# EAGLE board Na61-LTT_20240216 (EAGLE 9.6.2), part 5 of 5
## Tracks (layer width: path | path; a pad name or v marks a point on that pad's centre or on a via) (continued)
S$4670 (continued)
  Bottom 0.152: -7.4,145 -7.6,144.8
S$4671
  Bottom 0.152: -7.6,144.8 -7.6,144
S$4672
  Bottom 0.152: -9.4,145 -9.2,144.8
S$4673
  Bottom 0.152: -9.2,144.8 -9.2,144
S$4674
  Bottom 0.152: -11.4,145 -10.8,144.4
S$4675
  Bottom 0.152: -10.8,144.4 -10.8,144
S$4676
  Bottom 0.152: -13.4,145 -12.4,144
S$4677
  Bottom 0.152: -15.4,145 -14.4,144
S$4678
  Bottom 0.152: -14.4,144 -14,144
S$4679
  Bottom 0.152: -17.4,145 -16.4,144
S$4680
  Bottom 0.152: -16.4,144 -15.6,144
S$4681
  Bottom 0.152: -14.6,139 -15.6,140
S$4682
  Bottom 0.152: -15.6,140 -17.2,140
S$4683
  Bottom 0.152: -16.6,139 -17.4,139
S$4684
  Bottom 0.152: -17.4,139 -18.4,140
S$4685
  Bottom 0.152: -18.4,140 -18.8,140
S$4686
  Bottom 0.152: -18.6,139 -19.4,139
S$4687
  Bottom 0.152: -19.4,139 -20.4,140
S$4688
  Bottom 0.152: -20.6,139 -21,139
S$4689
  Bottom 0.152: -21,139 -22,140
S$4690
  Bottom 0.152: -22.6,139 -23.6,140
S$4691
  Bottom 0.152: -24.6,139 -25.2,139.6
S$4692
  Bottom 0.152: -25.2,139.6 -25.2,140
S$4693
  Bottom 0.152: -15.6,143 -16.2,143
S$4694
  Bottom 0.152: -16.2,143 -17.2,144
S$4695
  Bottom 0.152: -17.2,144 -18,144
S$4696
  Bottom 0.152: -17.6,143 -18.2,143
S$4697
  Bottom 0.152: -18.2,143 -19.2,144
S$4698
  Bottom 0.152: -19.2,144 -19.6,144
S$4699
  Bottom 0.152: -19.6,143 -20.2,143
S$4700
  Bottom 0.152: -20.2,143 -21.2,144
S$4701
  Bottom 0.152: -21.6,143 -21.8,143
S$4702
  Bottom 0.152: -21.8,143 -22.8,144
S$4703
  Bottom 0.152: -23.6,143 -24.4,143.8
S$4704
  Bottom 0.152: -24.4,143.8 -24.4,144
S$4705
  Bottom 0.152: 0.4,143 1,143
S$4706
  Bottom 0.152: 1,143 2,144
S$4707
  Bottom 0.152: 2.4,143 2.6,143
S$4708
  Bottom 0.152: 2.6,143 3.6,144
S$4709
  Bottom 0.152: 4.4,143 5.2,143.8
S$4710
  Bottom 0.152: 5.2,143.8 5.2,144
S$4711
  Bottom 0.152: 6.4,143 6.8,143.4
S$4712
  Bottom 0.152: 6.8,143.4 6.8,144
S$4713
  Bottom 0.152: 8.4,143 8.4,144
S$4714
  Bottom 0.152: -1.6,143 -0.6,143
S$4715
  Bottom 0.152: -0.6,143 0.4,144
S$4716
  Bottom 0.152: -0.6,139 0.4,140
S$4717
  Bottom 0.152: 0.4,140 1.2,140
S$4718
  Bottom 0.152: 1.4,139 1.8,139
S$4719
  Bottom 0.152: 1.8,139 2.8,140
S$4720
  Bottom 0.152: 3.4,139 4.4,140
S$4721
  Bottom 0.152: 5.4,139 6,139.6
S$4722
  Bottom 0.152: 6,139.6 6,140
S$4723
  Bottom 0.152: 7.4,139 7.6,139.2
S$4724
  Bottom 0.152: 7.6,139.2 7.6,140
S$4725
  Bottom 0.152: 9.4,139 9.2,139.2
S$4726
  Bottom 0.152: 9.2,139.2 9.2,140
S$4727
  Bottom 0.152: 11.4,139 10.8,139.6
S$4728
  Bottom 0.152: 10.8,139.6 10.8,140
S$4729
  Bottom 0.152: 13.4,139 12.4,140
S$4730
  Bottom 0.152: 15.4,139 15,139
S$4731
  Bottom 0.152: 15,139 14,140
S$4732
  Bottom 0.152: 17.4,139 16.6,139
S$4733
  Bottom 0.152: 16.6,139 15.6,140
S$4734
  Bottom 0.152: 10.4,143 10,143.4
S$4735
  Bottom 0.152: 10,143.4 10,144
S$4736
  Bottom 0.152: 12.4,143 11.6,143.8
S$4737
  Bottom 0.152: 11.6,143.8 11.6,144
S$4738
  Bottom 0.152: 14.4,143 14.2,143
S$4739
  Bottom 0.152: 14.2,143 13.2,144
S$4740
  Bottom 0.152: 16.4,143 15.8,143
S$4741
  Bottom 0.152: 15.8,143 14.8,144
S$4742
  Bottom 0.152: 18.4,141 17.4,140
S$4743
  Bottom 0.152: 17.4,140 16.4,140
S$4744
  Bottom 0.152: 16.6,145 17.2,145
S$4745
  Bottom 0.152: 17.2,145 18.2,144
S$4746
  Bottom 0.152: 18.2,144 18.8,144
S$4747
  Bottom 0.152: 18.6,145 19.6,144
S$4748
  Bottom 0.152: 19.6,144 20.4,144
S$4749
  Bottom 0.152: 20.6,145 21.6,144
S$4750
  Bottom 0.152: 21.6,144 22,144
S$4751
  Bottom 0.152: 22.6,145 23.6,144
S$4752
  Bottom 0.152: 24.6,145 25.2,144.4
S$4753
  Bottom 0.152: 25.2,144.4 25.2,144
S$4754
  Bottom 0.152: 15.6,149 16.6,148
S$4755
  Bottom 0.152: 16.6,148 18,148
S$4756
  Bottom 0.152: 17.6,149 18,149
S$4757
  Bottom 0.152: 18,149 19,148
S$4758
  Bottom 0.152: 19,148 19.6,148
S$4759
  Bottom 0.152: 19.6,149 20.2,149
S$4760
  Bottom 0.152: 20.2,149 21.2,148
S$4761
  Bottom 0.152: 21.6,149 21.8,149
S$4762
  Bottom 0.152: 21.8,149 22.8,148
S$4763
  Bottom 0.152: 23.6,149 24.4,148.2
S$4764
  Bottom 0.152: 24.4,148.2 24.4,148
S$4765
  Bottom 0.152: 17.2,144 16,144
S$4766
  Bottom 0.152: 16,144 15,145
S$4767
  Bottom 0.152: 15,145 14.6,145
S$4768
  Bottom 0.152: 50.8,143 50.2,143
S$4769
  Bottom 0.152: 50.2,143 49.2,144
S$4770
  Bottom 0.152: 48.8,143 48.6,143
S$4771
  Bottom 0.152: 48.6,143 47.6,144
S$4772
  Bottom 0.152: 46.8,143 46,143.8
S$4773
  Bottom 0.152: 46,143.8 46,144
S$4774
  Bottom 0.152: 44.8,143 44.4,143.4
S$4775
  Bottom 0.152: 44.4,143.4 44.4,144
S$4776
  Bottom 0.152: 42.8,143 42.8,144
S$4777
  Bottom 0.152: 52.8,143 51.8,143
S$4778
  Bottom 0.152: 51.8,143 50.8,144
S$4779
  Bottom 0.152: 51.8,139 50.8,140
S$4780
  Bottom 0.152: 50.8,140 50,140
S$4781
  Bottom 0.152: 49.8,139 49.4,139
S$4782
  Bottom 0.152: 49.4,139 48.4,140
S$4783
  Bottom 0.152: 47.8,139 46.8,140
S$4784
  Bottom 0.152: 45.8,139 45.2,139.6
S$4785
  Bottom 0.152: 45.2,139.6 45.2,140
S$4786
  Bottom 0.152: 43.8,139 43.6,139.2
S$4787
  Bottom 0.152: 43.6,139.2 43.6,140
S$4788
  Bottom 0.152: 41.8,139 42,139.2
S$4789
  Bottom 0.152: 42,139.2 42,140
S$4790
  Bottom 0.152: 39.8,139 40.4,139.6
S$4791
  Bottom 0.152: 40.4,139.6 40.4,140
S$4792
  Bottom 0.152: 37.8,139 38.8,140
S$4793
  Bottom 0.152: 35.8,139 36.2,139
S$4794
  Bottom 0.152: 36.2,139 37.2,140
S$4795
  Bottom 0.152: 33.8,139 34.6,139
S$4796
  Bottom 0.152: 34.6,139 35.6,140
S$4797
  Bottom 0.152: 40.8,143 41.2,143.4
S$4798
  Bottom 0.152: 41.2,143.4 41.2,144
S$4799
  Bottom 0.152: 38.8,143 39.6,143.8
S$4800
  Bottom 0.152: 39.6,143.8 39.6,144
S$4801
  Bottom 0.152: 36.8,143 37,143
S$4802
  Bottom 0.152: 37,143 38,144
S$4803
  Bottom 0.152: 34.8,143 35.4,143
S$4804
  Bottom 0.152: 35.4,143 36.4,144
S$4805
  Bottom 0.152: 32.8,141 33.8,140
S$4806
  Bottom 0.152: 33.8,140 34.8,140
S$4807
  Bottom 0.152: 34.6,145 34,145
S$4808
  Bottom 0.152: 34,145 33,144
S$4809
  Bottom 0.152: 33,144 32.4,144
S$4810
  Bottom 0.152: 32.6,145 31.6,144
S$4811
  Bottom 0.152: 31.6,144 30.8,144
S$4812
  Bottom 0.152: 30.6,145 29.6,144
S$4813
  Bottom 0.152: 29.6,144 29.2,144
S$4814
  Bottom 0.152: 28.6,145 27.6,144
S$4815
  Bottom 0.152: 26.6,145 26,144.4
S$4816
  Bottom 0.152: 26,144.4 26,144
S$4817
  Bottom 0.152: 35.6,149 34.6,148
S$4818
  Bottom 0.152: 34.6,148 33.2,148
S$4819
  Bottom 0.152: 33.6,149 33.2,149
S$4820
  Bottom 0.152: 33.2,149 32.2,148
S$4821
  Bottom 0.152: 32.2,148 31.6,148
S$4822
  Bottom 0.152: 31.6,149 31,149
S$4823
  Bottom 0.152: 31,149 30,148
S$4824
  Bottom 0.152: 29.6,149 29.4,149
S$4825
  Bottom 0.152: 29.4,149 28.4,148
S$4826
  Bottom 0.152: 27.6,149 26.8,148.2
S$4827
  Bottom 0.152: 26.8,148.2 26.8,148
S$4828
  Bottom 0.152: 34,144 35.2,144
S$4829
  Bottom 0.152: 35.2,144 36.2,145
S$4830
  Bottom 0.152: 36.2,145 36.6,145
S$4831  (2 unrouted)
  Top 0.813: 65,148.5 65,139.5
  Top 1.8: 66,145.5 64,145.5 | 66,148.5 65,148.5 64,148.5 | 66,142.5 64,142.5 | 66,139.5 65,139.5 64,139.5
S$4832
  Top 1.778: -104.08,140.82 -104.08,142.35
S$4833
  Top 1.778: -104.08,145.65 -104.08,147.18
S$4834
  Top 1.778: -99,140.82 -99,142.35
S$4835
  Top 1.778: -99,145.65 -99,147.18
S$4836
  Top 1.778: -93.92,140.82 -93.92,142.35
S$4837
  Top 1.778: -93.92,145.65 -93.92,147.18
S$4838
  Top 1.778: 93.92,140.82 93.92,142.35
S$4839
  Top 1.778: 93.92,145.65 93.92,147.18
S$4840
  Top 1.778: 99,140.82 99,142.35
S$4841
  Top 1.778: 99,145.65 99,147.18
S$4842
  Top 1.778: 104.08,140.82 104.08,142.35
S$4843
  Top 1.778: 104.08,145.65 104.08,147.18
S$4844  (via drill 0.2)
  other vias: -25.6,150.4
S$4845  (via drill 0.2)
  other vias: -8.6,137.6
S$4846  (via drill 0.2)
  other vias: 8.6,150.4
S$4847  (via drill 0.2)
  other vias: 25.6,137.6
S$4848  (via drill 0.2)
  other vias: 41.6,150.4
S$4849  (via drill 0.2)
  other vias: 52.8,150.4
S$4850  (via drill 0.2)
  other vias: -41.6,137.6
S$4851  (via drill 0.2)
  other vias: -52.8,137.6
S$4852
  Bottom 0.8: 9.4,156.9 9.4,155.1
S$4853
  Bottom 0.8: 11.4,156.9 11.4,155.1
S$4854
  Bottom 0.8: 8.4,159.1 8.4,160.9
S$4855
  Bottom 0.8: 10.4,159.1 10.4,160.9
S$4856
  Bottom 0.8: 5.4,156.9 5.4,155.1
S$4857
  Bottom 0.8: 7.4,156.9 7.4,155.1
S$4858
  Bottom 0.8: 6.4,159.1 6.4,160.9
S$4859
  Bottom 0.8: 4.4,159.1 4.4,160.9
S$4860
  Bottom 0.8: 3.4,156.9 3.4,155.1
S$4861
  Bottom 0.8: 1.4,156.9 1.4,155.1
S$4862
  Bottom 0.8: 2.4,159.1 2.4,160.9
S$4863
  Bottom 0.8: 0.4,159.1 0.4,160.9
S$4864
  Bottom 0.8: -0.6,156.9 -0.6,155.1
S$4865
  Bottom 0.8: -2.6,156.9 -2.6,155.1
S$4866
  Bottom 0.8: -1.6,159.1 -1.6,160.9
S$4867
  Bottom 0.8: 17.4,156.9 17.4,155.1
S$4868
  Bottom 0.8: 19.4,156.9 19.4,155.1
S$4869
  Bottom 0.8: 16.4,159.1 16.4,160.9
S$4870
  Bottom 0.8: 18.4,159.1 18.4,160.9
S$4871
  Bottom 0.8: 13.4,156.9 13.4,155.1
S$4872
  Bottom 0.8: 15.4,156.9 15.4,155.1
S$4873
  Bottom 0.8: 12.4,159.1 12.4,160.9
S$4874
  Bottom 0.8: 14.4,159.1 14.4,160.9
S$4875
  Bottom 0.8: -7.4,164.9 -7.4,163.1
S$4876
  Bottom 0.8: -5.4,164.9 -5.4,163.1
S$4877
  Bottom 0.8: -8.4,167.1 -8.4,168.9
S$4878
  Bottom 0.8: -6.4,167.1 -6.4,168.9
S$4879
  Bottom 0.8: -11.4,164.9 -11.4,163.1
S$4880
  Bottom 0.8: -9.4,164.9 -9.4,163.1
S$4881
  Bottom 0.8: -10.4,167.1 -10.4,168.9
S$4882
  Bottom 0.8: -12.4,167.1 -12.4,168.9
S$4883
  Bottom 0.8: -13.4,164.9 -13.4,163.1
S$4884
  Bottom 0.8: -15.4,164.9 -15.4,163.1
S$4885
  Bottom 0.8: -14.4,167.1 -14.4,168.9
S$4886
  Bottom 0.8: -16.4,167.1 -16.4,168.9
S$4887
  Bottom 0.8: -17.4,164.9 -17.4,163.1
S$4888
  Bottom 0.8: -19.4,164.9 -19.4,163.1
S$4889
  Bottom 0.8: -18.4,167.1 -18.4,168.9
S$4890
  Bottom 0.8: 0.6,164.9 0.6,163.1
S$4891
  Bottom 0.8: 2.6,164.9 2.6,163.1
S$4892
  Bottom 0.8: -0.4,167.1 -0.4,168.9
S$4893
  Bottom 0.8: 1.6,167.1 1.6,168.9
S$4894
  Bottom 0.8: -3.4,164.9 -3.4,163.1
S$4895
  Bottom 0.8: -1.4,164.9 -1.4,163.1
S$4896
  Bottom 0.8: -4.4,167.1 -4.4,168.9
S$4897
  Bottom 0.8: -2.4,167.1 -2.4,168.9
S$4898
  Bottom 0.8: -24.6,156.9 -24.6,155.1
S$4899
  Bottom 0.8: -22.6,156.9 -22.6,155.1
S$4900
  Bottom 0.8: -25.6,159.1 -25.6,160.9
S$4901
  Bottom 0.8: -23.6,159.1 -23.6,160.9
S$4902
  Bottom 0.8: -28.6,156.9 -28.6,155.1
S$4903
  Bottom 0.8: -26.6,156.9 -26.6,155.1
S$4904
  Bottom 0.8: -27.6,159.1 -27.6,160.9
S$4905
  Bottom 0.8: -29.6,159.1 -29.6,160.9
S$4906
  Bottom 0.8: -30.6,156.9 -30.6,155.1
S$4907
  Bottom 0.8: -32.6,156.9 -32.6,155.1
S$4908
  Bottom 0.8: -31.6,159.1 -31.6,160.9
S$4909
  Bottom 0.8: -33.6,159.1 -33.6,160.9
S$4910
  Bottom 0.8: -34.6,156.9 -34.6,155.1
S$4911
  Bottom 0.8: -36.6,156.9 -36.6,155.1
S$4912
  Bottom 0.8: -35.6,159.1 -35.6,160.9
S$4913
  Bottom 0.8: -16.6,156.9 -16.6,155.1
S$4914
  Bottom 0.8: -14.6,156.9 -14.6,155.1
S$4915
  Bottom 0.8: -17.6,159.1 -17.6,160.9
S$4916
  Bottom 0.8: -15.6,159.1 -15.6,160.9
S$4917
  Bottom 0.8: -20.6,156.9 -20.6,155.1
S$4918
  Bottom 0.8: -18.6,156.9 -18.6,155.1
S$4919
  Bottom 0.8: -21.6,159.1 -21.6,160.9
S$4920
  Bottom 0.8: -19.6,159.1 -19.6,160.9
S$4921
  Bottom 0.8: 26.6,164.9 26.6,163.1
S$4922
  Bottom 0.8: 28.6,164.9 28.6,163.1
S$4923
  Bottom 0.8: 25.6,167.1 25.6,168.9
S$4924
  Bottom 0.8: 27.6,167.1 27.6,168.9
S$4925
  Bottom 0.8: 22.6,164.9 22.6,163.1
S$4926
  Bottom 0.8: 24.6,164.9 24.6,163.1
S$4927
  Bottom 0.8: 23.6,167.1 23.6,168.9
S$4928
  Bottom 0.8: 21.6,167.1 21.6,168.9
S$4929
  Bottom 0.8: 20.6,164.9 20.6,163.1
S$4930
  Bottom 0.8: 18.6,164.9 18.6,163.1
S$4931
  Bottom 0.8: 19.6,167.1 19.6,168.9
S$4932
  Bottom 0.8: 17.6,167.1 17.6,168.9
S$4933
  Bottom 0.8: 16.6,164.9 16.6,163.1
S$4934
  Bottom 0.8: 14.6,164.9 14.6,163.1
S$4935
  Bottom 0.8: 15.6,167.1 15.6,168.9
S$4936
  Bottom 0.8: 34.6,164.9 34.6,163.1
S$4937
  Bottom 0.8: 36.6,164.9 36.6,163.1
S$4938
  Bottom 0.8: 33.6,167.1 33.6,168.9
S$4939
  Bottom 0.8: 35.6,167.1 35.6,168.9
S$4940
  Bottom 0.8: 30.6,164.9 30.6,163.1
S$4941
  Bottom 0.8: 32.6,164.9 32.6,163.1
S$4942
  Bottom 0.8: 29.6,167.1 29.6,168.9
S$4943
  Bottom 0.8: 31.6,167.1 31.6,168.9
S$4944
  Bottom 0.8: -41.8,164.9 -41.8,163.1
S$4945
  Bottom 0.8: -39.8,164.9 -39.8,163.1
S$4946
  Bottom 0.8: -42.8,167.1 -42.8,168.9
S$4947
  Bottom 0.8: -40.8,167.1 -40.8,168.9
S$4948
  Bottom 0.8: -45.8,164.9 -45.8,163.1
S$4949
  Bottom 0.8: -43.8,164.9 -43.8,163.1
S$4950
  Bottom 0.8: -44.8,167.1 -44.8,168.9
S$4951
  Bottom 0.8: -46.8,167.1 -46.8,168.9
S$4952
  Bottom 0.8: -47.8,164.9 -47.8,163.1
S$4953
  Bottom 0.8: -49.8,164.9 -49.8,163.1
S$4954
  Bottom 0.8: -48.8,167.1 -48.8,168.9
S$4955
  Bottom 0.8: -50.8,167.1 -50.8,168.9
S$4956
  Bottom 0.8: -51.8,164.9 -51.8,163.1
S$4957
  Bottom 0.8: -53.8,164.9 -53.8,163.1
S$4958
  Bottom 0.8: -52.8,167.1 -52.8,168.9
S$4959
  Bottom 0.8: -33.8,164.9 -33.8,163.1
S$4960
  Bottom 0.8: -31.8,164.9 -31.8,163.1
S$4961
  Bottom 0.8: -34.8,167.1 -34.8,168.9
S$4962
  Bottom 0.8: -32.8,167.1 -32.8,168.9
S$4963
  Bottom 0.8: -37.8,164.9 -37.8,163.1
S$4964
  Bottom 0.8: -35.8,164.9 -35.8,163.1
S$4965
  Bottom 0.8: -38.8,167.1 -38.8,168.9
S$4966
  Bottom 0.8: -36.8,167.1 -36.8,168.9
S$4967
  Bottom 0.8: 43.8,156.9 43.8,155.1
S$4968
  Bottom 0.8: 45.8,156.9 45.8,155.1
S$4969
  Bottom 0.8: 42.8,159.1 42.8,160.9
S$4970
  Bottom 0.8: 44.8,159.1 44.8,160.9
S$4971
  Bottom 0.8: 39.8,156.9 39.8,155.1
S$4972
  Bottom 0.8: 41.8,156.9 41.8,155.1
S$4973
  Bottom 0.8: 40.8,159.1 40.8,160.9
S$4974
  Bottom 0.8: 38.8,159.1 38.8,160.9
S$4975
  Bottom 0.8: 37.8,156.9 37.8,155.1
S$4976
  Bottom 0.8: 35.8,156.9 35.8,155.1
S$4977
  Bottom 0.8: 36.8,159.1 36.8,160.9
S$4978
  Bottom 0.8: 34.8,159.1 34.8,160.9
S$4979
  Bottom 0.8: 33.8,156.9 33.8,155.1
S$4980
  Bottom 0.8: 31.8,156.9 31.8,155.1
S$4981
  Bottom 0.8: 32.8,159.1 32.8,160.9
S$4982
  Bottom 0.8: 51.8,156.9 51.8,155.1
S$4983
  Bottom 0.8: 53.8,156.9 53.8,155.1
S$4984
  Bottom 0.8: 50.8,159.1 50.8,160.9
S$4985
  Bottom 0.8: 52.8,159.1 52.8,160.9
S$4986
  Bottom 0.8: 47.8,156.9 47.8,155.1
S$4987
  Bottom 0.8: 49.8,156.9 49.8,155.1
S$4988
  Bottom 0.8: 46.8,159.1 46.8,160.9
S$4989
  Bottom 0.8: 48.8,159.1 48.8,160.9
S$4990  (via drill 0.2)
  other vias: -50.8,166
S$4991  (via drill 0.2)
  other vias: -49.2,166
S$4992  (via drill 0.2)
  other vias: -47.6,166
S$4993  (via drill 0.2)
  other vias: -46,166
S$4994  (via drill 0.2)
  other vias: -44.4,166
S$4995  (via drill 0.2)
  other vias: -42.8,166
S$4996  (via drill 0.2)
  other vias: -41.2,166
S$4997  (via drill 0.2)
  other vias: -39.6,166
S$4998  (via drill 0.2)
  other vias: -38,166
S$4999  (via drill 0.2)
  other vias: -36.4,166
S$5000  (via drill 0.2)
  other vias: -34.8,166
S$5001  (via drill 0.2)
  other vias: -50,162
S$5002  (via drill 0.2)
  other vias: -48.4,162
S$5003  (via drill 0.2)
  other vias: -46.8,162
S$5004  (via drill 0.2)
  other vias: -45.2,162
S$5005  (via drill 0.2)
  other vias: -43.6,162
S$5006  (via drill 0.2)
  other vias: -42,162
S$5007  (via drill 0.2)
  other vias: -40.4,162
S$5008  (via drill 0.2)
  other vias: -38.8,162
S$5009  (via drill 0.2)
  other vias: -37.2,162
S$5010  (via drill 0.2)
  other vias: -35.6,162
S$5011  (via drill 0.2)
  other vias: -34,158
S$5012  (via drill 0.2)
  other vias: -32.4,158
S$5013  (via drill 0.2)
  other vias: -30.8,158
S$5014  (via drill 0.2)
  other vias: -29.2,158
S$5015  (via drill 0.2)
  other vias: -27.6,158
S$5016  (via drill 0.2)
  other vias: -33.2,162
S$5017  (via drill 0.2)
  other vias: -31.6,162
S$5018  (via drill 0.2)
  other vias: -30,162
S$5019  (via drill 0.2)
  other vias: -28.4,162
S$5020  (via drill 0.2)
  other vias: -26.8,162
S$5021  (via drill 0.2)
  other vias: -26,158
S$5022  (via drill 0.2)
  other vias: -0.4,166
S$5023  (via drill 0.2)
  other vias: -2,166
S$5024  (via drill 0.2)
  other vias: -3.6,166
S$5025  (via drill 0.2)
  other vias: -5.2,166
S$5026  (via drill 0.2)
  other vias: -6.8,166
S$5027  (via drill 0.2)
  other vias: -8.4,166
S$5028  (via drill 0.2)
  other vias: -10,166
S$5029  (via drill 0.2)
  other vias: -11.6,166
S$5030  (via drill 0.2)
  other vias: -13.2,166
S$5031  (via drill 0.2)
  other vias: -14.8,166
S$5032  (via drill 0.2)
  other vias: -16.4,166
S$5033  (via drill 0.2)
  other vias: -1.2,162
S$5034  (via drill 0.2)
  other vias: -2.8,162
S$5035  (via drill 0.2)
  other vias: -4.4,162
S$5036  (via drill 0.2)
  other vias: -6,162
S$5037  (via drill 0.2)
  other vias: -7.6,162
S$5038  (via drill 0.2)
  other vias: -9.2,162
S$5039  (via drill 0.2)
  other vias: -10.8,162
S$5040  (via drill 0.2)
  other vias: -12.4,162
S$5041  (via drill 0.2)
  other vias: -14,162
S$5042  (via drill 0.2)
  other vias: -15.6,162
S$5043  (via drill 0.2)
  other vias: -17.2,158
S$5044  (via drill 0.2)
  other vias: -18.8,158
S$5045  (via drill 0.2)
  other vias: -20.4,158
S$5046  (via drill 0.2)
  other vias: -22,158
S$5047  (via drill 0.2)
  other vias: -23.6,158
S$5048  (via drill 0.2)
  other vias: -18,162
S$5049  (via drill 0.2)
  other vias: -19.6,162
S$5050  (via drill 0.2)
  other vias: -21.2,162
S$5051  (via drill 0.2)
  other vias: -22.8,162
S$5052  (via drill 0.2)
  other vias: -24.4,162
S$5053  (via drill 0.2)
  other vias: -25.2,158
S$5054  (via drill 0.2)
  other vias: 0.4,162
S$5055  (via drill 0.2)
  other vias: 2,162
S$5056  (via drill 0.2)
  other vias: 3.6,162
S$5057  (via drill 0.2)
  other vias: 5.2,162
S$5058  (via drill 0.2)
  other vias: 6.8,162
S$5059  (via drill 0.2)
  other vias: 8.4,162
S$5060  (via drill 0.2)
  other vias: 10,162
S$5061  (via drill 0.2)
  other vias: 11.6,162
S$5062  (via drill 0.2)
  other vias: 13.2,162
S$5063  (via drill 0.2)
  other vias: 14.8,162
S$5064  (via drill 0.2)
  other vias: 16.4,158
S$5065  (via drill 0.2)
  other vias: 1.2,158
S$5066  (via drill 0.2)
  other vias: 2.8,158
S$5067  (via drill 0.2)
  other vias: 4.4,158
S$5068  (via drill 0.2)
  other vias: 6,158
S$5069  (via drill 0.2)
  other vias: 7.6,158
S$5070  (via drill 0.2)
  other vias: 9.2,158
S$5071  (via drill 0.2)
  other vias: 10.8,158
S$5072  (via drill 0.2)
  other vias: 12.4,158
S$5073  (via drill 0.2)
  other vias: 14,158
S$5074  (via drill 0.2)
  other vias: 15.6,158
S$5075  (via drill 0.2)
  other vias: 17.2,162
S$5076  (via drill 0.2)
  other vias: 18.8,162
S$5077  (via drill 0.2)
  other vias: 20.4,162
S$5078  (via drill 0.2)
  other vias: 18,166
S$5079  (via drill 0.2)
  other vias: 19.6,166
S$5080  (via drill 0.2)
  other vias: 21.2,166
S$5081  (via drill 0.2)
  other vias: 22,162
S$5082  (via drill 0.2)
  other vias: 22.8,166
S$5083  (via drill 0.2)
  other vias: 23.6,162
S$5084  (via drill 0.2)
  other vias: 24.4,166
S$5085  (via drill 0.2)
  other vias: 25.2,162
S$5086  (via drill 0.2)
  other vias: 50.8,162
S$5087  (via drill 0.2)
  other vias: 49.2,162
S$5088  (via drill 0.2)
  other vias: 47.6,162
S$5089  (via drill 0.2)
  other vias: 46,162
S$5090  (via drill 0.2)
  other vias: 44.4,162
S$5091  (via drill 0.2)
  other vias: 42.8,162
S$5092  (via drill 0.2)
  other vias: 41.2,162
S$5093  (via drill 0.2)
  other vias: 39.6,162
S$5094  (via drill 0.2)
  other vias: 38,162
S$5095  (via drill 0.2)
  other vias: 36.4,162
S$5096  (via drill 0.2)
  other vias: 34.8,158
S$5097  (via drill 0.2)
  other vias: 50,158
S$5098  (via drill 0.2)
  other vias: 48.4,158
S$5099  (via drill 0.2)
  other vias: 46.8,158
S$5100  (via drill 0.2)
  other vias: 45.2,158
S$5101  (via drill 0.2)
  other vias: 43.6,158
S$5102  (via drill 0.2)
  other vias: 42,158
S$5103  (via drill 0.2)
  other vias: 40.4,158
S$5104  (via drill 0.2)
  other vias: 38.8,158
S$5105  (via drill 0.2)
  other vias: 37.2,158
S$5106  (via drill 0.2)
  other vias: 35.6,158
S$5107  (via drill 0.2)
  other vias: 34,162
S$5108  (via drill 0.2)
  other vias: 32.4,162
S$5109  (via drill 0.2)
  other vias: 30.8,162
S$5110  (via drill 0.2)
  other vias: 33.2,166
S$5111  (via drill 0.2)
  other vias: 31.6,166
S$5112  (via drill 0.2)
  other vias: 30,166
S$5113  (via drill 0.2)
  other vias: 29.2,162
S$5114  (via drill 0.2)
  other vias: 28.4,166
S$5115  (via drill 0.2)
  other vias: 27.6,162
S$5116  (via drill 0.2)
  other vias: 26.8,166
S$5117  (via drill 0.2)
  other vias: 26,162
S$5118
  Bottom 0.152: -52.8,167 -51.8,166
S$5119
  Bottom 0.152: -51.8,166 -50.8,166
S$5120
  Bottom 0.152: -50.8,167 -50.2,167
S$5121
  Bottom 0.152: -50.2,167 -49.2,166
S$5122
  Bottom 0.152: -48.8,167 -48.6,167
S$5123
  Bottom 0.152: -48.6,167 -47.6,166
S$5124
  Bottom 0.152: -46.8,167 -46,166.2
S$5125
  Bottom 0.152: -46,166.2 -46,166
S$5126
  Bottom 0.152: -44.8,167 -44.4,166.6
S$5127
  Bottom 0.152: -44.4,166.6 -44.4,166
S$5128
  Bottom 0.152: -42.8,167 -42.8,166
S$5129
  Bottom 0.152: -40.8,167 -41.2,166.6
S$5130
  Bottom 0.152: -41.2,166.6 -41.2,166
S$5131
  Bottom 0.152: -38.8,167 -39.6,166.2
S$5132
  Bottom 0.152: -39.6,166.2 -39.6,166
S$5133
  Bottom 0.152: -36.8,167 -37,167
S$5134
  Bottom 0.152: -37,167 -38,166
S$5135
  Bottom 0.152: -34.8,167 -35.4,167
S$5136
  Bottom 0.152: -35.4,167 -36.4,166
S$5137
  Bottom 0.152: -32.8,167 -33.8,166
S$5138
  Bottom 0.152: -33.8,166 -34.8,166
S$5139
  Bottom 0.152: -51.8,163 -50.8,162
S$5140
  Bottom 0.152: -50.8,162 -50,162
S$5141
  Bottom 0.152: -49.8,163 -48.8,162
S$5142
  Bottom 0.152: -48.8,162 -48.4,162
S$5143
  Bottom 0.152: -47.8,163 -46.8,162
S$5144
  Bottom 0.152: -45.8,163 -45.2,162.4
S$5145
  Bottom 0.152: -45.2,162.4 -45.2,162
S$5146
  Bottom 0.152: -43.8,163 -43.6,162.8
S$5147
  Bottom 0.152: -43.6,162.8 -43.6,162
S$5148
  Bottom 0.152: -41.8,163 -42,162.8
S$5149
  Bottom 0.152: -42,162.8 -42,162
S$5150
  Bottom 0.152: -39.8,163 -40.4,162.4
S$5151
  Bottom 0.152: -40.4,162.4 -40.4,162
S$5152
  Bottom 0.152: -37.8,163 -38.8,162
S$5153
  Bottom 0.152: -35.8,163 -36.8,162
S$5154
  Bottom 0.152: -36.8,162 -37.2,162
S$5155
  Bottom 0.152: -33.8,163 -34.8,162
S$5156
  Bottom 0.152: -34.8,162 -35.6,162
S$5157
  Bottom 0.152: -36.6,157 -35.6,158
S$5158
  Bottom 0.152: -35.6,158 -34,158
S$5159
  Bottom 0.152: -34.6,157 -33.8,157
S$5160
  Bottom 0.152: -33.8,157 -32.8,158
S$5161
  Bottom 0.152: -32.8,158 -32.4,158
S$5162
  Bottom 0.152: -32.6,157 -31.8,157
S$5163
  Bottom 0.152: -31.8,157 -30.8,158
S$5164
  Bottom 0.152: -30.6,157 -30.2,157
S$5165
  Bottom 0.152: -30.2,157 -29.2,158
S$5166
  Bottom 0.152: -28.6,157 -27.6,158
S$5167
  Bottom 0.152: -26.6,157 -26,157.6
S$5168
  Bottom 0.152: -26,157.6 -26,158
S$5169
  Bottom 0.152: -35.6,161 -35,161
S$5170
  Bottom 0.152: -35,161 -34,162
S$5171
  Bottom 0.152: -34,162 -33.2,162
S$5172
  Bottom 0.152: -33.6,161 -33,161
S$5173
  Bottom 0.152: -33,161 -32,162
S$5174
  Bottom 0.152: -32,162 -31.6,162
S$5175
  Bottom 0.152: -31.6,161 -31,161
S$5176
  Bottom 0.152: -31,161 -30,162
S$5177
  Bottom 0.152: -29.6,161 -29.4,161
S$5178
  Bottom 0.152: -29.4,161 -28.4,162
S$5179
  Bottom 0.152: -27.6,161 -26.8,161.8
S$5180
  Bottom 0.152: -26.8,161.8 -26.8,162
S$5181
  Bottom 0.152: 1.6,167 0.6,166
S$5182
  Bottom 0.152: 0.6,166 -0.4,166
S$5183
  Bottom 0.152: -0.4,167 -1,167
S$5184
  Bottom 0.152: -1,167 -2,166
S$5185
  Bottom 0.152: -2.4,167 -2.6,167
S$5186
  Bottom 0.152: -2.6,167 -3.6,166
S$5187
  Bottom 0.152: -4.4,167 -5.2,166.2
S$5188
  Bottom 0.152: -5.2,166.2 -5.2,166
S$5189
  Bottom 0.152: -6.4,167 -6.8,166.6
S$5190
  Bottom 0.152: -6.8,166.6 -6.8,166
S$5191
  Bottom 0.152: -8.4,167 -8.4,166
S$5192
  Bottom 0.152: -10.4,167 -10,166.6
S$5193
  Bottom 0.152: -10,166.6 -10,166
S$5194
  Bottom 0.152: -12.4,167 -11.6,166.2
S$5195
  Bottom 0.152: -11.6,166.2 -11.6,166
S$5196
  Bottom 0.152: -14.4,167 -14.2,167
S$5197
  Bottom 0.152: -14.2,167 -13.2,166
S$5198
  Bottom 0.152: -16.4,167 -15.8,167
S$5199
  Bottom 0.152: -15.8,167 -14.8,166
S$5200
  Bottom 0.152: -18.4,167 -17.4,166
S$5201
  Bottom 0.152: -17.4,166 -16.4,166
S$5202
  Bottom 0.152: 0.6,163 -0.4,162
S$5203
  Bottom 0.152: -0.4,162 -1.2,162
S$5204
  Bottom 0.152: -1.4,163 -2.4,162
S$5205
  Bottom 0.152: -2.4,162 -2.8,162
S$5206
  Bottom 0.152: -3.4,163 -4.4,162
S$5207
  Bottom 0.152: -5.4,163 -6,162.4
S$5208
  Bottom 0.152: -6,162.4 -6,162
S$5209
  Bottom 0.152: -7.4,163 -7.6,162.8
S$5210
  Bottom 0.152: -7.6,162.8 -7.6,162
S$5211
  Bottom 0.152: -9.4,163 -9.2,162.8
S$5212
  Bottom 0.152: -9.2,162.8 -9.2,162
S$5213
  Bottom 0.152: -11.4,163 -10.8,162.4
S$5214
  Bottom 0.152: -10.8,162.4 -10.8,162
S$5215
  Bottom 0.152: -13.4,163 -12.4,162
S$5216
  Bottom 0.152: -15.4,163 -14.4,162
S$5217
  Bottom 0.152: -14.4,162 -14,162
S$5218
  Bottom 0.152: -17.4,163 -16.4,162
S$5219
  Bottom 0.152: -16.4,162 -15.6,162
S$5220
  Bottom 0.152: -14.6,157 -15.6,158
S$5221
  Bottom 0.152: -15.6,158 -17.2,158
S$5222
  Bottom 0.152: -16.6,157 -17.4,157
S$5223
  Bottom 0.152: -17.4,157 -18.4,158
S$5224
  Bottom 0.152: -18.4,158 -18.8,158
S$5225
  Bottom 0.152: -18.6,157 -19.4,157
S$5226
  Bottom 0.152: -19.4,157 -20.4,158
S$5227
  Bottom 0.152: -20.6,157 -21,157
S$5228
  Bottom 0.152: -21,157 -22,158
S$5229
  Bottom 0.152: -22.6,157 -23.6,158
S$5230
  Bottom 0.152: -24.6,157 -25.2,157.6
S$5231
  Bottom 0.152: -25.2,157.6 -25.2,158
S$5232
  Bottom 0.152: -15.6,161 -16.2,161
S$5233
  Bottom 0.152: -16.2,161 -17.2,162
S$5234
  Bottom 0.152: -17.2,162 -18,162
S$5235
  Bottom 0.152: -17.6,161 -18.2,161
S$5236
  Bottom 0.152: -18.2,161 -19.2,162
S$5237
  Bottom 0.152: -19.2,162 -19.6,162
S$5238
  Bottom 0.152: -19.6,161 -20.2,161
S$5239
  Bottom 0.152: -20.2,161 -21.2,162
S$5240
  Bottom 0.152: -21.6,161 -21.8,161
S$5241
  Bottom 0.152: -21.8,161 -22.8,162
S$5242
  Bottom 0.152: -23.6,161 -24.4,161.8
S$5243
  Bottom 0.152: -24.4,161.8 -24.4,162
S$5244
  Bottom 0.152: 0.4,161 1,161
S$5245
  Bottom 0.152: 1,161 2,162
S$5246
  Bottom 0.152: 2.4,161 2.6,161
S$5247
  Bottom 0.152: 2.6,161 3.6,162
S$5248
  Bottom 0.152: 4.4,161 5.2,161.8
S$5249
  Bottom 0.152: 5.2,161.8 5.2,162
S$5250
  Bottom 0.152: 6.4,161 6.8,161.4
S$5251
  Bottom 0.152: 6.8,161.4 6.8,162
S$5252
  Bottom 0.152: 8.4,161 8.4,162
S$5253
  Bottom 0.152: -1.6,161 -0.6,161
S$5254
  Bottom 0.152: -0.6,161 0.4,162
S$5255
  Bottom 0.152: -0.6,157 0.4,158
S$5256
  Bottom 0.152: 0.4,158 1.2,158
S$5257
  Bottom 0.152: 1.4,157 1.8,157
S$5258
  Bottom 0.152: 1.8,157 2.8,158
S$5259
  Bottom 0.152: 3.4,157 4.4,158
S$5260
  Bottom 0.152: 5.4,157 6,157.6
S$5261
  Bottom 0.152: 6,157.6 6,158
S$5262
  Bottom 0.152: 7.4,157 7.6,157.2
S$5263
  Bottom 0.152: 7.6,157.2 7.6,158
S$5264
  Bottom 0.152: 9.4,157 9.2,157.2
S$5265
  Bottom 0.152: 9.2,157.2 9.2,158
S$5266
  Bottom 0.152: 11.4,157 10.8,157.6
S$5267
  Bottom 0.152: 10.8,157.6 10.8,158
S$5268
  Bottom 0.152: 13.4,157 12.4,158
S$5269
  Bottom 0.152: 15.4,157 15,157
S$5270
  Bottom 0.152: 15,157 14,158
S$5271
  Bottom 0.152: 17.4,157 16.6,157
S$5272
  Bottom 0.152: 16.6,157 15.6,158
S$5273
  Bottom 0.152: 10.4,161 10,161.4
S$5274
  Bottom 0.152: 10,161.4 10,162
S$5275
  Bottom 0.152: 12.4,161 11.6,161.8
S$5276
  Bottom 0.152: 11.6,161.8 11.6,162
S$5277
  Bottom 0.152: 14.4,161 14.2,161
S$5278
  Bottom 0.152: 14.2,161 13.2,162
S$5279
  Bottom 0.152: 16.4,161 15.8,161
S$5280
  Bottom 0.152: 15.8,161 14.8,162
S$5281
  Bottom 0.152: 18.4,159 17.4,158
S$5282
  Bottom 0.152: 17.4,158 16.4,158
S$5283
  Bottom 0.152: 16.6,163 17.2,163
S$5284
  Bottom 0.152: 17.2,163 18.2,162
S$5285
  Bottom 0.152: 18.2,162 18.8,162
S$5286
  Bottom 0.152: 18.6,163 19.6,162
S$5287
  Bottom 0.152: 19.6,162 20.4,162
S$5288
  Bottom 0.152: 20.6,163 21.6,162
S$5289
  Bottom 0.152: 21.6,162 22,162
S$5290
  Bottom 0.152: 22.6,163 23.6,162
S$5291
  Bottom 0.152: 24.6,163 25.2,162.4
S$5292
  Bottom 0.152: 25.2,162.4 25.2,162
S$5293
  Bottom 0.152: 15.6,167 16.6,166
S$5294
  Bottom 0.152: 16.6,166 18,166
S$5295
  Bottom 0.152: 17.6,167 18,167
S$5296
  Bottom 0.152: 18,167 19,166
S$5297
  Bottom 0.152: 19,166 19.6,166
S$5298
  Bottom 0.152: 19.6,167 20.2,167
S$5299
  Bottom 0.152: 20.2,167 21.2,166
S$5300
  Bottom 0.152: 21.6,167 21.8,167
S$5301
  Bottom 0.152: 21.8,167 22.8,166
S$5302
  Bottom 0.152: 23.6,167 24.4,166.2
S$5303
  Bottom 0.152: 24.4,166.2 24.4,166
S$5304
  Bottom 0.152: 17.2,162 16,162
S$5305
  Bottom 0.152: 16,162 15,163
S$5306
  Bottom 0.152: 15,163 14.6,163
S$5307
  Bottom 0.152: 50.8,161 50.2,161
S$5308
  Bottom 0.152: 50.2,161 49.2,162
S$5309
  Bottom 0.152: 48.8,161 48.6,161
S$5310
  Bottom 0.152: 48.6,161 47.6,162
S$5311
  Bottom 0.152: 46.8,161 46,161.8
S$5312
  Bottom 0.152: 46,161.8 46,162
S$5313
  Bottom 0.152: 44.8,161 44.4,161.4
S$5314
  Bottom 0.152: 44.4,161.4 44.4,162
S$5315
  Bottom 0.152: 42.8,161 42.8,162
S$5316
  Bottom 0.152: 52.8,161 51.8,161
S$5317
  Bottom 0.152: 51.8,161 50.8,162
S$5318
  Bottom 0.152: 51.8,157 50.8,158
S$5319
  Bottom 0.152: 50.8,158 50,158
S$5320
  Bottom 0.152: 49.8,157 49.4,157
S$5321
  Bottom 0.152: 49.4,157 48.4,158
S$5322
  Bottom 0.152: 47.8,157 46.8,158
S$5323
  Bottom 0.152: 45.8,157 45.2,157.6
S$5324
  Bottom 0.152: 45.2,157.6 45.2,158
S$5325
  Bottom 0.152: 43.8,157 43.6,157.2
S$5326
  Bottom 0.152: 43.6,157.2 43.6,158
S$5327
  Bottom 0.152: 41.8,157 42,157.2
S$5328
  Bottom 0.152: 42,157.2 42,158
S$5329
  Bottom 0.152: 39.8,157 40.4,157.6
S$5330
  Bottom 0.152: 40.4,157.6 40.4,158
S$5331
  Bottom 0.152: 37.8,157 38.8,158
S$5332
  Bottom 0.152: 35.8,157 36.2,157
S$5333
  Bottom 0.152: 36.2,157 37.2,158
S$5334
  Bottom 0.152: 33.8,157 34.6,157
S$5335
  Bottom 0.152: 34.6,157 35.6,158
S$5336
  Bottom 0.152: 40.8,161 41.2,161.4
S$5337
  Bottom 0.152: 41.2,161.4 41.2,162
S$5338
  Bottom 0.152: 38.8,161 39.6,161.8
S$5339
  Bottom 0.152: 39.6,161.8 39.6,162
S$5340
  Bottom 0.152: 36.8,161 37,161
S$5341
  Bottom 0.152: 37,161 38,162
S$5342
  Bottom 0.152: 34.8,161 35.4,161
S$5343
  Bottom 0.152: 35.4,161 36.4,162
S$5344
  Bottom 0.152: 32.8,159 33.8,158
S$5345
  Bottom 0.152: 33.8,158 34.8,158
S$5346
  Bottom 0.152: 34.6,163 34,163
S$5347
  Bottom 0.152: 34,163 33,162
S$5348
  Bottom 0.152: 33,162 32.4,162
S$5349
  Bottom 0.152: 32.6,163 31.6,162
S$5350
  Bottom 0.152: 31.6,162 30.8,162
S$5351
  Bottom 0.152: 30.6,163 29.6,162
S$5352
  Bottom 0.152: 29.6,162 29.2,162
S$5353
  Bottom 0.152: 28.6,163 27.6,162
S$5354
  Bottom 0.152: 26.6,163 26,162.4
S$5355
  Bottom 0.152: 26,162.4 26,162
S$5356
  Bottom 0.152: 35.6,167 34.6,166
S$5357
  Bottom 0.152: 34.6,166 33.2,166
S$5358
  Bottom 0.152: 33.6,167 33.2,167
S$5359
  Bottom 0.152: 33.2,167 32.2,166
S$5360
  Bottom 0.152: 32.2,166 31.6,166
S$5361
  Bottom 0.152: 31.6,167 31,167
S$5362
  Bottom 0.152: 31,167 30,166
S$5363
  Bottom 0.152: 29.6,167 29.4,167
S$5364
  Bottom 0.152: 29.4,167 28.4,166
S$5365
  Bottom 0.152: 27.6,167 26.8,166.2
S$5366
  Bottom 0.152: 26.8,166.2 26.8,166
S$5367
  Bottom 0.152: 34,162 35.2,162
S$5368
  Bottom 0.152: 35.2,162 36.2,163
S$5369
  Bottom 0.152: 36.2,163 36.6,163
S$5370
  Top 0.813: 65,166.5 65,157.5
  Top 1.8: 66,166.5 65,166.5 64,166.5 | 66,157.5 65,157.5 64,157.5
S$5371
  Top 1.778: -104.08,158.82 -104.08,160.35
S$5372
  Top 1.778: -104.08,163.65 -104.08,165.18
S$5373
  Top 1.778: -99,158.82 -99,160.35
S$5374
  Top 1.778: -99,163.65 -99,165.18
S$5375
  Top 1.778: -93.92,158.82 -93.92,160.35
S$5376
  Top 1.778: -93.92,163.65 -93.92,165.18
S$5377
  Top 1.778: 93.92,158.82 93.92,160.35
S$5378
  Top 1.778: 93.92,163.65 93.92,165.18
S$5379
  Top 1.778: 99,158.82 99,160.35
S$5380
  Top 1.778: 99,163.65 99,165.18
S$5381
  Top 1.778: 104.08,158.82 104.08,160.35
S$5382
  Top 1.778: 104.08,163.65 104.08,165.18
S$5383  (via drill 0.2)
  other vias: -25.6,168.4
S$5384  (via drill 0.2)
  other vias: -8.6,155.6
S$5385  (via drill 0.2)
  other vias: 8.6,168.4
S$5386  (via drill 0.2)
  other vias: 25.6,155.6
S$5387  (via drill 0.2)
  other vias: 41.6,168.4
S$5388  (via drill 0.2)
  other vias: 52.8,168.4
S$5389  (via drill 0.2)
  other vias: -41.6,155.6
S$5390  (via drill 0.2)
  other vias: -52.8,155.6
S$5391
  Top 0.813: -93.92,-1.5 -93.92,1
S$5392
  Top 0.813: -93.92,16.5 -93.92,19
S$5393
  Top 0.61: -65,21 -65,16.5 | -65,16.5 -65,15 | -65,16.5 -68.5,16.5 -70,18
  Top 0.813: -70,18 -93.5,18
  Top 1.8: -64,21 -65,21 -66,21 | -64,15 -65,15 -66,15
S$5394
  Top 0.813: -93.92,34.5 -93.92,37
S$5395  (1 unrouted)
  Top 0.61: -65,39 -65,34.5 | -65,34.5 -65,33 | -65,34.5 -68.5,34.5 -70,36
  Top 0.813: -70,36 -93.5,36
  Top 1.8: -64,36 -66,36 | -64,39 -65,39 -66,39 | -64,33 -65,33 -66,33
S$5396
  Top 0.813: -93.92,52.5 -93.92,55
S$5397  (1 unrouted)
  Top 0.61: -65,57 -65,52.5 | -65,52.5 -65,51 | -65,52.5 -68.5,52.5 -70,54
  Top 0.813: -70,54 -93.5,54
  Top 1.8: -64,54 -66,54 | -64,57 -65,57 -66,57 | -64,51 -65,51 -66,51
S$5398
  Top 0.813: -93.92,70.5 -93.92,73
S$5399  (1 unrouted)
  Top 0.61: -65,75 -65,70.5 | -65,70.5 -65,69 | -65,70.5 -68.5,70.5 -70,72
  Top 0.813: -70,72 -93.5,72
  Top 1.8: -64,72 -66,72 | -64,75 -65,75 -66,75 | -64,69 -65,69 -66,69
S$5400
  Top 0.813: -93.92,88.5 -93.92,91
S$5401  (1 unrouted)
  Top 0.61: -65,93 -65,88.5 | -65,88.5 -65,87 | -65,88.5 -68.5,88.5 -70,90
  Top 0.813: -70,90 -93.5,90
  Top 1.8: -64,90 -66,90 | -64,93 -65,93 -66,93 | -64,87 -65,87 -66,87
S$5402
  Top 0.813: -93.92,106.5 -93.92,109
S$5403  (1 unrouted)
  Top 0.61: -65,111 -65,106.5 | -65,106.5 -65,105 | -65,106.5 -68.5,106.5 -70,108
  Top 0.813: -70,108 -93.5,108
  Top 1.8: -64,108 -66,108 | -64,111 -65,111 -66,111 | -64,105 -65,105 -66,105
S$5404
  Top 0.813: -93.92,124.5 -93.92,127
S$5405  (1 unrouted)
  Top 0.61: -65,129 -65,124.5 | -65,124.5 -65,123 | -65,124.5 -68.5,124.5 -70,126
  Top 0.813: -70,126 -93.5,126
  Top 1.8: -64,126 -66,126 | -64,129 -65,129 -66,129 | -64,123 -65,123 -66,123
S$5406
  Top 0.813: -93.92,142.5 -93.92,145
S$5407
  Top 0.61: -65,147 -65,142.5 | -65,142.5 -65,141 | -65,142.5 -68.5,142.5 -70,144
  Top 0.813: -70,144 -93.5,144
  Top 1.8: -64,147 -65,147 -66,147 | -64,141 -65,141 -66,141
S$5408
  Top 0.813: -93.92,160.5 -93.92,163
S$5409
  Top 3: 1.5,178 -1.5,178
S$5410
  Top 2: -28,178 -30,178
S$5411
  Top 2: 23,178 21,178
S$5412
  Top 2: 107,180 105,180
S$5413
  Top 0.813: -98,180 -90,180 -88,182 -74,182 -70,178 -50,178 -44,178
S$5414
  Top 3: -96.5,180 -99.5,180
S$5415
  Top 0.813: -125,-16 -118,-16 -115,-19 -69,-19 -67,-21 -43,-21 -38,-16 56,-16
S$5416
  Top 3: -126.5,135 -129.5,135
S$5417  (2 unrouted)
  Bottom 2: -159,124 -157,124 | -159,2 -157,2 | -159,38 -157,38
S$5418
  Top 0.813: -128,176 -128,164
S$5419
  Top 3: -126.5,27 -129.5,27
S$5420
  Top 0.813: -130,35 -128,35 | -128,35 -126,35 -128,35 | -128,35 -128,27
  Top 2: -126,35 -126,33 | -129,35 -130,35 -131,35
S$5421
  Top 0.813: -126,48 -122.5,48
S$5422  (via drill 4.2)
  other vias: -99,189
S$5423  (via drill 4.2)
  other vias: -99,-27
S$5424  (via drill 4.2)
  other vias: -117,-27
S$5425  (via drill 4.2)
  other vias: -135,-27
S$5426
  Top 2: 107,174 105,174
S$5427  (via drill 4.2)
  other vias: -153,-27
S$5428  (via drill 4.2)
  other vias: 99,-27
S$5429  (via drill 4.2)
  other vias: 117,-27
S$5430  (via drill 4.2)
  other vias: 117,-9
S$5431  (via drill 4.2)
  other vias: 99,189
S$5432  (via drill 4.2)
  other vias: 117,189
S$5433  (via drill 4.2)
  other vias: 117,99
S$5434
  Top 0.813: -99,164 -99,-3
S$5435
  Top 0.813: -128,128 -128,135 -122,135
S$5436
  Top 2: -145,164 -147,164
S$5437
  Top 3: -126.5,171 -129.5,171
S$5438
  Top 2: -128,176 -126,176
S$5439
  Top 0.813: 92,-16 92,-12 99,-6 99,-2
  Top 2: 92,-16 90,-16
S$5440  (via drill 4.2)
  other vias: -135,189
S$5441
  Top 3: -123.5,-16 -126.5,-16
S$5442
  Top 0.508: 106,174 104,174
  Top 0.813: 104,174 99,167 99,165
S$5443
  Top 0.813: 65.1,18 93.9,18
S$5444
  Top 0.813: 93.9,20 93.9,16
S$5445
  Top 3: -123.5,-8 -126.5,-8
S$5446
  Top 3: -54.5,-16 -57.5,-16
S$5447
  Top 0.813: 65.1,36 93.9,36
S$5448
  Top 0.813: 93.9,38 93.9,34
S$5449
  Top 0.813: 65.1,54 93.9,54
S$5450
  Top 0.813: 93.9,56 93.9,52
S$5451
  Top 0.813: 65.1,72 93.9,72
S$5452
  Top 0.813: 93.9,74 93.9,70
S$5453
  Top 0.813: 65.1,90 93.9,90
S$5454
  Top 0.813: 93.9,92 93.9,88
S$5455
  Top 0.813: 65.1,108 93.9,108
S$5456
  Top 0.813: 93.9,110 93.9,106
S$5457
  Top 0.813: 65.1,126 93.9,126
S$5458
  Top 0.813: 93.9,128 93.9,124
S$5459
  Top 0.813: 65.1,144 93.9,144
S$5460
  Top 0.813: 93.9,146 93.9,142
S$5461
  Top 0.813: 65.1,162 93.9,162
S$5462
  Top 0.813: 93.9,164 93.9,160
S$5463
  Top 0.813: 65.1,0 93.9,0
S$5464
  Top 0.813: 93.9,2 93.9,-2
S$5465
  Top 0.813: -122,150 -122,151 -120,153 -99,153
S$5466
  Top 0.813: 2,178 7,178
S$5467
  Top 0.813: 106,180 116,180
S$5468
  Top 2: -7,178 -9,178
S$5469
  Top 0.813: -8,178 -2,178
S$5470
  Top 0.813: -112,176 -110,176 -108,174 -90,174 -86,178 -76,178 -72,174 71,174 75,178 85,178 89,174 93,174
S$5471  (via drill 4.2)
  other vias: -153,189
S$5472  (via drill 4.2)
  other vias: -117,189
S$5473  (4 unrouted)
  Bottom 2: -159,160 -157,160 | 98,163.25 100,163.25 | 98,160.75 100,160.75 | 98,158.25 100,158.25 | 98,165.75 100,165.75
S$5474  (via drill 4.2)
  other vias: -153,153
S$5475  (via drill 4.2)
  other vias: -153,117
S$5476
  Top 2: -122,150 -122,148
S$5477  (via drill 4.2)
  other vias: -153,81
S$5478  (via drill 4.2)
  other vias: -153,45
S$5479  (via drill 4.2)
  other vias: -153,9
S$5480
  Top 2: -147,35 -149,35
S$5481
  Top 2: -126,49 -126,47
S$5482
  Top 3: -122.5,49.5 -122.5,46.5
S$5483
  Top 2: 110,-16 108,-16
S$5484  (via drill 4.2)
  other vias: 117,9
S$5485  (via drill 4.2)
  other vias: 117,45
S$5486  (via drill 4.2)
  other vias: 117,27
S$5487  (via drill 4.2)
  other vias: 117,63
S$5488  (via drill 4.2)
  other vias: 117,171
S$5489  (via drill 4.2)
  other vias: 117,117
S$5490  (via drill 4.2)
  other vias: 117,81
S$5491  (via drill 4.2)
  other vias: 117,135
S$5492  (via drill 4.2)
  other vias: 117,153
S$5493
  Top 3: 57.5,-16 54.5,-16
S$5494  (2 unrouted)
  Top 0.813: 65,4.5 65,-4.5
  Top 1.8: 66,-1.5 64,-1.5 | 66,1.5 64,1.5 | 66,4.5 65,4.5 64,4.5 | 66,-4.5 65,-4.5 64,-4.5
S$5495
  Top 1.8: -64,0 -66,0
S$5496
  Top 1.8: -64,18 -66,18
S$5497
  Top 2: 93,174 91,174
S$5498
  Top 2: 93,180 91,180
S$5499
  Top 0.508: 90,180 93,180
  Top 0.813: 43,178 68,178 72,182 88,182 90,180
S$5500
  Top 2: 9,178 7,178
S$5501  (1 unrouted)
  Top 2: 44,178 42,178
  Top 3: 52.5,178 49.5,178
S$5502
  Top 0.813: 23,178 28,178
S$5503
  Top 2: 30,178 28,178
S$5504  (1 unrouted)
  Top 0.813: 99,164 99,-3 | 104,164 104,-3
S$5505
  Top 1.8: 66,163.5 64,163.5
S$5506
  Top 1.8: 66,160.5 64,160.5
S$5507
  Top 0.61: -65,165 -65,160.5 | -65,160.5 -65,159 | -65,160.5 -68.5,160.5 -70,162
  Top 0.813: -70,162 -93.5,162
  Top 1.8: -64,159 -65,159 -66,159 | -64,165 -65,165 -66,165
S$5508
  Top 2: -42,178 -44,178
S$5509
  Top 0.813: -29,178 -23,178
S$5510
  Top 3: -49.5,178 -52.5,178
S$5511
  Top 2: -21,178 -23,178
S$5512
  Top 2: -145,128 -147,128
S$5513
  Top 2: -127,128 -129,128
S$5514
  Top 2: -122,136 -122,134
S$5515
  Top 2: -114,176 -112,176
S$5516
  Top 2: -127,164 -129,164
S$5517
  Top 0.813: -122,-8 -118,-8 -111,-15 -66,-15 -65,-16 -56,-16
S$5518
  Top 1.8: -64,162 -66,162
S$5519
  Top 1.8: -64,144 -66,144
S$5520  (3 unrouted)
  Bottom 2: 98,127.25 100,127.25 | 98,124.75 100,124.75 | 98,122.25 100,122.25 | 98,129.75 100,129.75
S$5521  (3 unrouted)
  Bottom 2: -136,163.25 -134,163.25 | -136,160.75 -134,160.75 | -136,158.25 -134,158.25 | -136,165.75 -134,165.75
S$5522  (3 unrouted)
  Bottom 2: -136,127.25 -134,127.25 | -136,124.75 -134,124.75 | -136,122.25 -134,122.25 | -136,129.75 -134,129.75
S$5523  (3 unrouted)
  Bottom 2: 98,1.25 100,1.25 | 98,-1.25 100,-1.25 | 98,-3.75 100,-3.75 | 98,3.75 100,3.75
S$5524  (3 unrouted)
  Bottom 2: 98,37.25 100,37.25 | 98,34.75 100,34.75 | 98,32.25 100,32.25 | 98,39.75 100,39.75
S$5525  (3 unrouted)
  Bottom 2: -136,1.25 -134,1.25 | -136,-1.25 -134,-1.25 | -136,-3.75 -134,-3.75 | -136,3.75 -134,3.75
S$5526  (3 unrouted)
  Bottom 2: -136,37.25 -134,37.25 | -136,34.75 -134,34.75 | -136,32.25 -134,32.25 | -136,39.75 -134,39.75
S$5527  (via drill 0.2 pad 0.3)
  other vias: -72,-30
S$5528  (via drill 0.2 pad 0.3)
  other vias: -54,-30
S$5529  (via drill 0.2 pad 0.3)
  other vias: -36,-30
S$5530  (via drill 0.2 pad 0.3)
  other vias: -90,-30
S$5531  (via drill 0.2 pad 0.3)
  other vias: -108,-30
S$5532  (via drill 0.2 pad 0.3)
  other vias: -126,-30
S$5533  (via drill 0.2 pad 0.3)
  other vias: -144,-30
S$5534  (via drill 0.2 pad 0.3)
  other vias: -18,-30
S$5535  (via drill 0.2 pad 0.3)
  other vias: 0,-30
S$5536  (via drill 0.2 pad 0.3)
  other vias: 18,-30
S$5537  (via drill 0.2 pad 0.3)
  other vias: 36,-30
S$5538  (via drill 0.2 pad 0.3)
  other vias: 54,-30
S$5539  (via drill 0.2 pad 0.3)
  other vias: 72,-30
S$5540  (via drill 0.2 pad 0.3)
  other vias: 90,-30
S$5541  (via drill 0.2 pad 0.3)
  other vias: 108,-30
S$5542  (via drill 0.2 pad 0.3)
  other vias: -72,192
S$5543  (via drill 0.2 pad 0.3)
  other vias: -54,192
S$5544  (via drill 0.2 pad 0.3)
  other vias: -36,192
S$5545  (via drill 0.2 pad 0.3)
  other vias: -90,192
S$5546  (via drill 0.2 pad 0.3)
  other vias: -108,192
S$5547  (via drill 0.2 pad 0.3)
  other vias: -126,192
S$5548  (via drill 0.2 pad 0.3)
  other vias: -144,192
S$5549  (via drill 0.2 pad 0.3)
  other vias: -18,192
S$5550  (via drill 0.2 pad 0.3)
  other vias: 0,192
S$5551  (via drill 0.2 pad 0.3)
  other vias: 18,192
S$5552  (via drill 0.2 pad 0.3)
  other vias: 36,192
S$5553  (via drill 0.2 pad 0.3)
  other vias: 54,192
S$5554  (via drill 0.2 pad 0.3)
  other vias: 72,192
S$5555  (via drill 0.2 pad 0.3)
  other vias: 90,192
S$5556  (via drill 0.2 pad 0.3)
  other vias: 108,192
S$5557  (via drill 0.2 pad 0.3)
  other vias: 120,54
S$5558  (via drill 0.2 pad 0.3)
  other vias: 120,72
S$5559  (via drill 0.2 pad 0.3)
  other vias: 120,90
S$5560  (via drill 0.2 pad 0.3)
  other vias: 120,36
S$5561  (via drill 0.2 pad 0.3)
  other vias: 120,18
S$5562  (via drill 0.2 pad 0.3)
  other vias: 120,0
S$5563  (via drill 0.2 pad 0.3)
  other vias: 120,-18
S$5564  (via drill 0.2 pad 0.3)
  other vias: 120,108
S$5565  (via drill 0.2 pad 0.3)
  other vias: 120,126
S$5566  (via drill 0.2 pad 0.3)
  other vias: 120,144
S$5567  (via drill 0.2 pad 0.3)
  other vias: 120,162
S$5568  (via drill 0.2 pad 0.3)
  other vias: 120,180
S$5572  (via drill 0.2 pad 0.3)
  other vias: -156,54
S$5573  (via drill 0.2 pad 0.3)
  other vias: -156,72
S$5574  (via drill 0.2 pad 0.3)
  other vias: -156,90
S$5575  (via drill 0.2 pad 0.3)
  other vias: -156,36
S$5576  (via drill 0.2 pad 0.3)
  other vias: -156,18
S$5577  (via drill 0.2 pad 0.3)
  other vias: -156,0
S$5578  (via drill 0.2 pad 0.3)
  other vias: -156,-18
S$5579  (via drill 0.2 pad 0.3)
  other vias: -156,108
S$5580  (via drill 0.2 pad 0.3)
  other vias: -156,126
S$5581  (via drill 0.2 pad 0.3)
  other vias: -156,144
S$5582  (via drill 0.2 pad 0.3)
  other vias: -156,162
S$5583  (via drill 0.2 pad 0.3)
  other vias: -156,180
S$5601  (via drill 0.2 pad 0.3)
  other vias: 104,-2
S$5602  (via drill 0.2 pad 0.3)
  other vias: 104,2
S$5603  (via drill 0.2 pad 0.3)
  other vias: 104,16
S$5604  (via drill 0.2 pad 0.3)
  other vias: 104,20
S$5605  (via drill 0.2 pad 0.3)
  other vias: 104,34
S$5606  (via drill 0.2 pad 0.3)
  other vias: 104,38
S$5607  (via drill 0.2 pad 0.3)
  other vias: 104,52
S$5608  (via drill 0.2 pad 0.3)
  other vias: 104,56
S$5609  (via drill 0.2 pad 0.3)
  other vias: 104,70
S$5610  (via drill 0.2 pad 0.3)
  other vias: 104,74
S$5611  (via drill 0.2 pad 0.3)
  other vias: 104,88
S$5612  (via drill 0.2 pad 0.3)
  other vias: 104,92
S$5613  (via drill 0.2 pad 0.3)
  other vias: 104,106
S$5614  (via drill 0.2 pad 0.3)
  other vias: 104,110
S$5615  (via drill 0.2 pad 0.3)
  other vias: 104,124
S$5616  (via drill 0.2 pad 0.3)
  other vias: 104,128
S$5617  (via drill 0.2 pad 0.3)
  other vias: 104,142
S$5618  (via drill 0.2 pad 0.3)
  other vias: 104,146
S$5619  (via drill 0.2 pad 0.3)
  other vias: 104,160
S$5620  (via drill 0.2 pad 0.3)
  other vias: 104,164
S$5621  (via drill 0.2 pad 0.3)
  other vias: -104,-2
S$5622  (via drill 0.2 pad 0.3)
  other vias: -104,2
S$5623  (via drill 0.2 pad 0.3)
  other vias: -104,16
S$5624  (via drill 0.2 pad 0.3)
  other vias: -104,20
S$5625  (via drill 0.2 pad 0.3)
  other vias: -104,34
S$5626  (via drill 0.2 pad 0.3)
  other vias: -104,38
S$5627  (via drill 0.2 pad 0.3)
  other vias: -104,52
S$5628  (via drill 0.2 pad 0.3)
  other vias: -104,56
S$5629  (via drill 0.2 pad 0.3)
  other vias: -104,70
S$5630  (via drill 0.2 pad 0.3)
  other vias: -104,74
S$5631  (via drill 0.2 pad 0.3)
  other vias: -104,88
S$5632  (via drill 0.2 pad 0.3)
  other vias: -104,92
S$5633  (via drill 0.2 pad 0.3)
  other vias: -104,106
S$5634  (via drill 0.2 pad 0.3)
  other vias: -104,110
S$5635  (via drill 0.2 pad 0.3)
  other vias: -104,124
S$5636  (via drill 0.2 pad 0.3)
  other vias: -104,128
S$5637  (via drill 0.2 pad 0.3)
  other vias: -104,142
S$5638  (via drill 0.2 pad 0.3)
  other vias: -104,146
S$5639  (via drill 0.2 pad 0.3)
  other vias: -104,160
S$5640  (via drill 0.2 pad 0.3)
  other vias: -104,164
(copper drawn outside any net)
  shapes: Top area x1280

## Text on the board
tDocu: FieldW | Gnd | SkirtTop | SkirtBot | ZeroGrid | SenseW | Gas | Cathode | GatingG
THT: --R-- | --R-- | --R-- | --R-- | --R-- | --R-- | --R-- | --C-- | --R-- | --C-- | --R-- | --C-- | --C--
CageSupp: R6 / R12
Remarks: L:SkirtTop | L:FcBaseBot | Via:FcBaseBot | L:FcBaseTop | Hv:Cath / FcB-Cath | Hv:Cath / PadP-FcB | 00.0 / - 08.4 / 16.8 / - 25.6 / 34.4 / - 42.8 / 51.2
